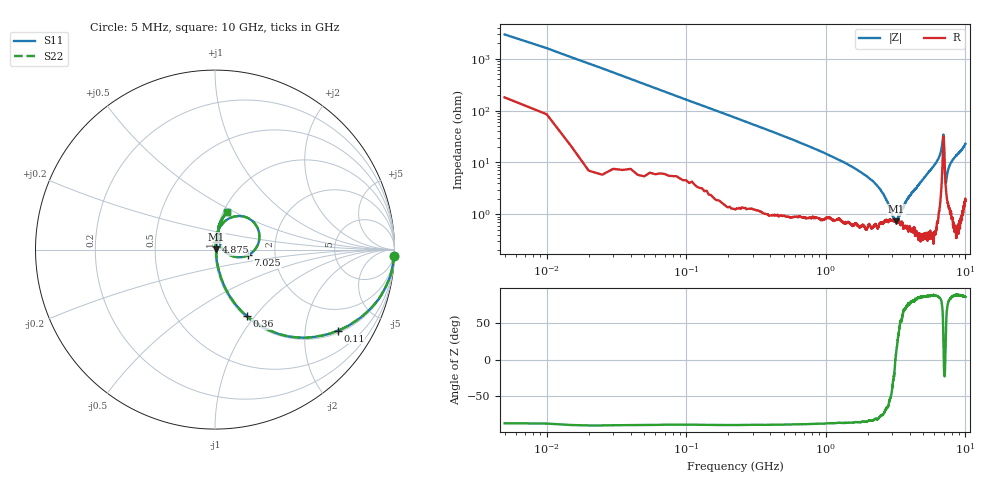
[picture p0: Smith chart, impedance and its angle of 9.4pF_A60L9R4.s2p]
! Amotech Co.,Ltd.
! http://www.amotech.co.kr/
! Part Number: A60L9R4
! These Parameters are Measured in Series Mode Connection
! Operation Temp=25[degC], DC Bias Voltage=0[V]
! Freq. Start=5[MHz] Stop=10[GHz], 2000[Steps]
! Date: Monday, July 14, 2020, 09:56:28
# GHZ S RI R 50.000000
!Freq.(Hz) S11(Real) S11(Imag) S21(Real) S21(Imag) S12(Real) S12(Imag) S22(Real) S22(Imag)
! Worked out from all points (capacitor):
!   2000 points, 5 MHz to 10 GHz, reference 50 ohm
!   read as one part in series: C = 9.75 pF near 55 MHz
!   lowest |Z| = 734 mohm at 3.205 GHz (marker M1)
!   series resonance near 3.152 GHz, so ESL is about 260 pH
!   S11 on the Smith chart (normalised r, x): 5 MHz: 5, -59; 110 MHz: 1.09, -2.97; 360 MHz: 1.02, -0.91; 4.875 GHz: 1.01, +0.09; 7.025 GHz: 1.44, -0.09; 10 GHz: 1.04, +0.46
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0.005  0.9968 -0.0336  0.00319 0.0336  0.00319 0.0336  0.9968 -0.0336
0.065  0.8576 -0.3375  0.1424 0.3375  0.1424 0.3375  0.8576 -0.3375
0.11  0.6829 -0.4512  0.3171 0.4512  0.3171 0.4512  0.6829 -0.4512
0.225  0.3498 -0.4685  0.6502 0.4685  0.6502 0.4685  0.3498 -0.4685
0.36  0.1758 -0.3694  0.8242 0.3694  0.8242 0.3694  0.1758 -0.3694
0.83  0.0405 -0.1757  0.9595 0.1757  0.9595 0.1757  0.0405 -0.1757
1.675  0.0115 -0.0705  0.9885 0.0705  0.9885 0.0705  0.0115 -0.0705
2.44  0.0077 -0.0297  0.9923 0.0297  0.9923 0.0297  0.0077 -0.0297
3.05  0.00751 -0.00394  0.9925 0.00394  0.9925 0.00394  0.00751 -0.00394
3.205  0.00707 0.00178  0.9929 -0.00178  0.9929 -0.00178  0.00707 0.00178
3.34  0.00775 0.0059  0.9923 -0.0059  0.9923 -0.0059  0.00775 0.0059
3.83  0.0063 0.0184  0.9937 -0.0184  0.9937 -0.0184  0.0063 0.0184
4.875  0.00575 0.0438  0.9942 -0.0438  0.9942 -0.0438  0.00575 0.0438
5.005  0.00598 0.0478  0.994 -0.0478  0.994 -0.0478  0.00598 0.0478
6.67  0.0458 0.1489  0.9542 -0.1489  0.9542 -0.1489  0.0458 0.1489
6.925  0.2152 0.1525  0.7848 -0.1525  0.7848 -0.1525  0.2152 0.1525
7.025  0.1826 -0.0317  0.8174 0.0317  0.8174 0.0317  0.1826 -0.0317
7.165  0.0483 -0.00447  0.9517 0.00447  0.9517 0.00447  0.0483 -0.00447
7.235  0.0329 0.0191  0.9671 -0.0191  0.9671 -0.0191  0.0329 0.0191
7.635  0.0191 0.0785  0.9809 -0.0785  0.9809 -0.0785  0.0191 0.0785
8.335  0.0195 0.1206  0.9805 -0.1206  0.9805 -0.1206  0.0195 0.1206
10  0.0669 0.2109  0.9331 -0.2109  0.9331 -0.2109  0.0669 0.2109
